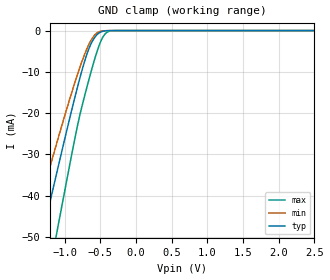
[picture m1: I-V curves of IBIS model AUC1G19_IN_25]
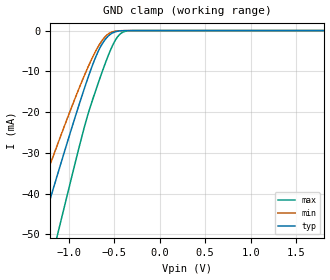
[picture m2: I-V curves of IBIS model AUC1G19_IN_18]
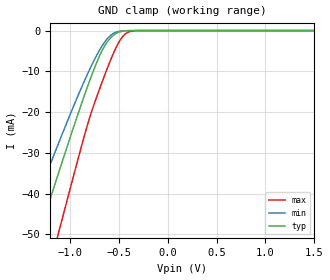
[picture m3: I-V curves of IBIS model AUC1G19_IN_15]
| TEXAS INSTRUMENTS INCORPORATED
| Standard Linear and Logic Group
| IBIS Model of SN74AUC1G19
| 1-of-2 DECORDER/MULTIPLEXER
| This file contains package information for the following:
|  SOT 6-pin (DBV) package as [Component] AUC1G19_DBV
|  SOT 6-pin (DCK) package as [Component] AUC1G19_DCK
|  DSBGA 6-pin (YEP_YZP) package as [Component] AUC1G19_YEP_YZP
| This device can be powered at the following Vccs:
|  2.5 volt Vcc
|  1.8 volt Vcc
|  1.5 volt Vcc
|  1.2 volt Vcc
|  0.8 volt Vcc
| This file provides unique models under the [Model Selector] for each Vcc.
| For operation at a specific Vcc, select the appropriate model after each
| [Model Selector] keyword.
[IBIS Ver]   3.2
[Comment char]  |_char
[File Name]   sn74auc1g19.ibs
[File Rev]   1.1 | x_die
[Date]   April 01, 2005
[Source]   Data created from TI-SPICE simulations at TI-SLL.
[Notes]   The following is an IBIS list for the AUC1G19.
   Please contact sllibis@ti.com with questions and
   comments concerning SLL IBIS models.
   - FILE REV HISTORY
   - 1.1 Release IBIS file on 04/02/05
   - Non-monotonic data in pullup and pulldown due to
   feedback circuit.
   - Power clamp data deleted as there is no power-clamp diode.
[Disclaimer] Property of Texas Instruments Incorporated.  Unauthorized
   reproduction and/or distribution is strictly prohibited.
   This product is protected under copyright law.
   Created  2005, (C) Copyright  2005, Texas Instruments
   Incorporated, All Rights Reserved
   UNLESS THERE IS A SIGNED, WRITTEN AGREEMENT TO THE
   CONTRARY, TEXAS INSTRUMENTS (TI) IS PROVIDING THE IBIS
   MODELS  AND WITHOUT ANY WARRANTY, EXPRESSED OR
   IMPLIED.  TI assumes no liability for:
   1) the accuracy of the IBIS models provided to your
   company;
   2) the proper functioning of these IBIS Models in your
   design or for any resulting applications; or
   3) infringement of patents, copyrights or intellectual
   property rights resulting from your use of these IBIS
   models.
   TI provides IBIS Models as a service to our customers.
   You and your company shall not distribute, sell or give
   these models to anyone else without prior written
   permission from TI.
   TI reserves the right to make changes to our products or
   to discontinue any semiconductor product or service
   without notice, and advises our customers to obtain the
   latest version of relevant information to verify, before
   placing orders, that the information being relied on is
   current.
   Please be aware that your receipt and use of the IBIS
   information provided shall serve as acceptance of these
   terms and conditions.  If you do not accept these terms,
   you should return or destroy the IBIS models and any
   other accompanying information immediately.
| Component AUC1G19_DBV 6-pin SOT
[Component]   AUC1G19_DBV
[Manufacturer]   Texas Instruments, Inc.
[Package]
|   typ   min   max
R_pkg   2.500e-02   1.900e-02   3.700e-02
L_pkg   1.524e-09   1.260e-09   1.751e-09
C_pkg   2.450e-13   1.980e-13   2.640e-13
[Pin]   signal_name   model_name   R_pin   L_pin   C_pin
1   A   AUC1G19_IN   2.100e-02   1.405e-09   2.460e-13
2   GND   GND   3.700e-02   1.751e-09   2.630e-13
3   EB   AUC1G19_IN   2.600e-02   1.493e-09   2.470e-13
4   Y1   AUC1G19_OUT   1.900e-02   1.620e-09   2.640e-13
5   VCC   POWER   2.400e-02   1.260e-09   1.980e-13
6   Y0   AUC1G19_OUT   2.100e-02   1.617e-09   2.500e-13
| Component AUC1G19_DCK 6-pin SOT
[Component]   AUC1G19_DCK
[Manufacturer]   Texas Instruments, Inc.
[Package]
|   typ   min   max
R_pkg   1.400e-02   1.100e-02   2.100e-02
L_pkg   9.480e-10   7.840e-10   1.103e-09
C_pkg   1.910e-13   1.670e-13   2.050e-13
[Pin]   signal_name   model_name   R_pin   L_pin   C_pin
1   A   AUC1G19_IN   1.300e-02   9.840e-10   1.960e-13
2   GND   GND   2.100e-02   1.103e-09   2.050e-13
3   EB   AUC1G19_IN   1.100e-02   9.980e-10   1.970e-13
4   Y1   AUC1G19_OUT   1.300e-02   9.040e-10   1.900e-13
5   VCC   POWER   1.500e-02   7.840e-10   1.670e-13
6   Y0   AUC1G19_OUT   1.200e-02   9.160e-10   1.950e-13
| Component AUC1G19_YEP_YZP 6-pin DSBGA
[Component]   AUC1G19_YEP_YZP
[Manufacturer]   Texas Instruments, Inc.
[Package]
|   typ   min   max
R_pkg   1.000e-03   1.000e-03   2.100e-02
L_pkg   2.450e-11   2.400e-11   1.103e-09
C_pkg   5.600e-14   0.000e+00   2.050e-13
[Pin]   signal_name   model_name   R_pin   L_pin   C_pin
1   A   AUC1G19_IN   1.000e-03   2.500e-11   6.400e-14
2   GND   GND   1.000e-03   2.400e-11   6.700e-14
3   EB   AUC1G19_IN   1.000e-03   2.500e-11   6.400e-14
4   Y1   AUC1G19_OUT   1.000e-03   2.500e-11   6.400e-14
5   VCC   POWER   1.000e-03   2.400e-11   6.700e-14
6   Y0   AUC1G19_OUT   1.000e-03   2.500e-11   6.400e-14
| Model AUC1G19_IN
[Model Selector]   AUC1G19_IN
AUC1G19_IN_25   2.5 volt Vcc
AUC1G19_IN_18   1.8 volt Vcc
AUC1G19_IN_15   1.5 volt Vcc
AUC1G19_IN_12   1.2 volt Vcc
AUC1G19_IN_08   0.8 volt Vcc
| Model AUC1G19_OUT
[Model Selector]   AUC1G19_OUT
AUC1G19_OUT_25   2.5 volt Vcc
AUC1G19_OUT_18   1.8 volt Vcc
AUC1G19_OUT_15   1.5 volt Vcc
AUC1G19_OUT_12   1.2 volt Vcc
AUC1G19_OUT_08   0.8 volt Vcc
| Models and submodels in the file (10): AUC1G19_IN_25 (Input), AUC1G19_IN_18 (Input), AUC1G19_IN_15 (Input), AUC1G19_IN_12 (Input), AUC1G19_IN_08 (Input), AUC1G19_OUT_25 (Output), AUC1G19_OUT_18 (Output), AUC1G19_OUT_15 (Output), AUC1G19_OUT_12 (Output), AUC1G19_OUT_08 (Output)
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[Model]   AUC1G19_IN_25
Model_type  Input
Vinl=0.7
Vinh=1.7
| variable   typ   min   max
C_comp   2.38pF   1.90pF   2.86pF
[Temperature Range]   40   100   -40
| Ambient temperature   25   85   -40
[Voltage range]   2.5   2.3   2.7
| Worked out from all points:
|   GND clamp passes 1 mA (typ) near -0.55 V on its own axis
[GND Clamp]
| AUC1G19_IN_25
|   Voltage   I(typ)   I(min)   I(max)
-3.6V     -226mA     -190mA     -273.7mA
-1.485V   -62.86mA   -50.58mA   -83.39mA
-1.435V   -59.04mA   -47.41mA   -78.83mA
-1.3V     -48.79mA   -38.95mA   -66.5mA
-1.115V   -34.91mA   -27.61mA   -49.58mA
-830mV    -14.47mA   -11.23mA   -24.01mA
-720mV    -7.514mA   -5.815mA   -15.91mA
-625mV    -3.068mA   -2.231mA   -9.764mA
-525mV    -682.5uA   -368.4uA   -4.063mA
-430mV    -73.19uA   -35.23uA   -779.9uA
-325mV    -3.339uA   -2.025uA   -30.75uA
2.5V      313.9pA    401.7pA    470.4pA
[Model]   AUC1G19_IN_18
Model_type  Input
Vinl=0.63
Vinh=1.17
| variable   typ   min   max
C_comp   2.45pF   1.99pF   2.86pF
[Temperature Range]   40   100   -40
| Ambient temperature   25   85   -40
[Voltage range]   1.8   1.65   1.95
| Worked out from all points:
|   GND clamp passes 1 mA (typ) near -0.55 V on its own axis
[GND Clamp]
| AUC1G19_IN_18
|   Voltage   I(typ)   I(min)   I(max)
-3.6V     -226mA     -190mA     -273.7mA
-1.485V   -62.86mA   -50.58mA   -83.39mA
-1.44V    -59.42mA   -47.73mA   -79.29mA
-1.305V   -49.17mA   -39.26mA   -66.96mA
-1.105V   -34.17mA   -27.01mA   -48.67mA
-830mV    -14.47mA   -11.23mA   -24.01mA
-685mV    -5.632mA   -4.335mA   -13.61mA
-565mV    -1.377mA   -850.6uA   -6.177mA
-490mV    -325.8uA   -161.4uA   -2.516mA
-425mV    -63.96uA   -30.9uA    -691.3uA
-300mV    -1.501uA   -996.5nA   -11.88uA
1.8V      203.2pA    298pA      235.5pA
[Model]   AUC1G19_IN_15
Model_type  Input
Vinl=0.525
Vinh=0.975
| variable   typ   min   max
C_comp   2.49pF   2.04pF   2.87pF
[Temperature Range]   40   100   -40
| Ambient temperature   25   85   -40
[Voltage range]   1.5   1.4   1.6
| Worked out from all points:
|   GND clamp passes 1 mA (typ) near -0.55 V on its own axis
[GND Clamp]
| AUC1G19_IN_15
|   Voltage   I(typ)   I(min)   I(max)
-3.6V     -226mA     -190mA     -273.7mA
-1.465V   -61.33mA   -49.31mA   -81.57mA
-1.33V    -51.06mA   -40.82mA   -69.24mA
-1.29V    -48.03mA   -38.33mA   -65.59mA
-1.125V   -35.66mA   -28.21mA   -50.49mA
-1.075V   -31.95mA   -25.21mA   -45.93mA
-815mV    -13.46mA   -10.44mA   -22.78mA
-695mV    -6.145mA   -4.742mA   -14.26mA
-575mV    -1.604mA   -1.024mA   -6.747mA
-435mV    -83.63uA   -40.14uA   -876.8uA
-310mV    -2.071uA   -1.325uA   -17.49uA
1.5V      165.9pA    259.3pA    172.1pA
